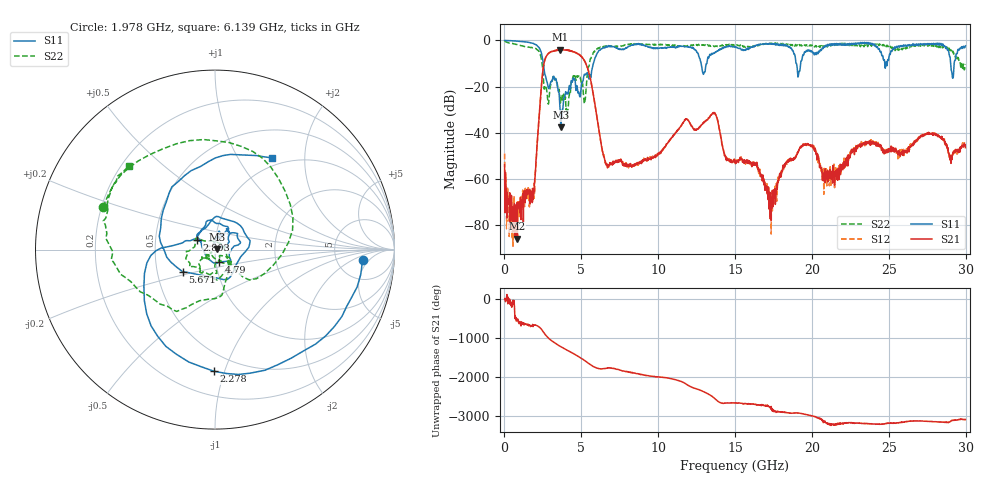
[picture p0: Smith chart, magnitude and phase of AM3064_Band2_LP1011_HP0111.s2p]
# Hz S DB R 50.0
!freq dBS11 angS11 dBS21 angS21 dBS12 angS12 dBS22 angS22
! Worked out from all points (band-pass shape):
!   1600 points, 10 MHz to 29.98 GHz, reference 50 ohm
!   highest |S21| = -4.01 dB at 3.628 GHz (marker M1); lowest = -85.7 dB at 797.2 MHz (marker M2)
!   |S21| within 3 dB of the highest: 2.711 GHz to 5.001 GHz (2.29 GHz wide, 59.4 % of centre)
!   lowest |S11| = -37.6 dB at 3.684 GHz (marker M3), VSWR 1.03, Z = 51.3 + j0.201 ohm
!   |S11| at or under -10 dB: 2.53 GHz to 5.779 GHz (3.249 GHz wide, 78.2 % of centre); 12.79 GHz to 13.16 GHz (366.2 MHz wide, 2.82 % of centre); 18.98 GHz to 19.27 GHz (289.1 MHz wide, 1.51 % of centre)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
!   |S22| runs from -32.9 to -0.2 dB; largest |S21 - S12| = 0.02
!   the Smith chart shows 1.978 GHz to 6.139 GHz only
!   S11 on the Smith chart (normalised r, x): 1.978 GHz: 9.09, -3.43; 2.278 GHz: 0.37, -0.92; 2.803 GHz: 0.81, +0.09; 4.79 GHz: 1.03, -0.14; 5.671 GHz: 0.68, -0.17; 6.139 GHz: 0.88, +1.40
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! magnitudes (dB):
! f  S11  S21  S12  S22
! 10 MHz  0.0  -53.7  -49.0  -0.2
! 797.2 MHz  -0.3  -85.7  -77.0  -1.8
! 1.978 GHz  -1.7  -59.8  -60.7  -3.5
! 2.278 GHz  -3.4  -30.7  -30.7  -5.1
! 2.803 GHz  -18.9  -6.1  -6.0  -25.1
! 3.628 GHz  -30.3  -4.0  -4.1  -26.2
! 3.684 GHz  -37.6  -4.1  -4.1  -24.1
! 4.79 GHz  -22.8  -5.9  -5.7  -15.6
! 5.015 GHz  -18.6  -7.2  -7.0  -18.7
! 5.671 GHz  -13.2  -19.4  -19.2  -7.2
! 6.139 GHz  -4.4  -38.6  -38.6  -3.5
! 6.739 GHz  -2.8  -54.2  -54.0  -2.3
! 10 GHz  -3.5  -48.7  -48.9  -1.9
! 13.6 GHz  -5.4  -31.8  -31.3  -2.5
! 15 GHz  -2.7  -52.3  -52.2  -1.9
! 17.33 GHz  -1.4  -70.4  -65.9  -1.4
! 19.99 GHz  -4.6  -45.7  -45.7  -2.0
! 20.82 GHz  -2.8  -56.9  -58.3  -2.4
! 25 GHz  -8.0  -48.3  -48.5  -2.2
! 28.39 GHz  -1.3  -42.1  -41.9  -3.1
! 29.18 GHz  -16.2  -48.6  -49.4  -4.8
! 29.98 GHz  -2.4  -46.4  -45.0  -10.3
